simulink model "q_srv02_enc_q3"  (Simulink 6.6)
settings: Solver=FixedStepDiscrete  StartTime=0.0  StopTime=inf  FixedStep=0.002  RelTol=1e-3  AbsTol=1e-6
undefined symbols (not defined in the file or in its folder): HIL, qc_get_step_size
libraries: quarc_library x3, simulink x1

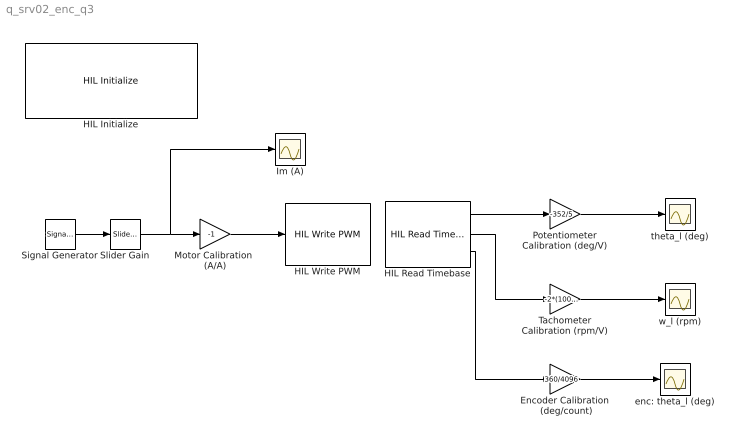
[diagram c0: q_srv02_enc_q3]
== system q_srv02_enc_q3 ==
  Encoder Calibration  (deg/count) : Gain  Gain=360/4096
  HIL Initialize : quarc_library/Data Acquisition/Generic/Configuration/HIL Initialize  object_name=HIL-1  board_type=q3_controlpaq_fw  board_number=0  exclusive=off  active=on  hardware_clocks=[]  clock_modes=[]  set_clock_params_at_start=off  set_clock_params_at_switch_in=off  analog_input_channels=0:1  analog_input_maximums=10  analog_input_minimums=-10  set_analog_input_params_at_start=off  set_analog_input_params_at_switch_in=off  analog_output_channels=[]  analog_output_maximums=[]  analog_output_minimums=[]  initial_analog_outputs=[]  final_analog_outputs=[]  watchdog_analog_outputs=[]  set_analog_output_params_at_start=off  set_analog_output_params_at_switch_in=off  set_analog_outputs_at_start=off  set_analog_outputs_at_switch_in=off  set_analog_outputs_at_terminate=off  set_analog_outputs_at_switch_out=off  set_analog_outputs_on_watchdog=off  digital_input_channels=[0:1]  digital_output_channels=[0]  digital_output_configuration=[]  initial_digital_outputs=0  final_digital_outputs=0  watchdog_digital_outputs=[]  set_digital_output_params_at_start=off  set_digital_output_params_at_switch_in=off  set_digital_outputs_at_start=on  set_digital_outputs_at_switch_in=off  set_digital_outputs_at_terminate=on  set_digital_outputs_at_switch_out=off  set_digital_outputs_on_watchdog=off  encoder_channels=0:2  quadrature=[]  encoder_filter_frequency=[]  initial_encoder_counts=0  set_encoder_params_at_start=off  set_encoder_params_at_switch_in=off  set_encoder_counts_at_start=on  set_encoder_counts_at_switch_in=off  pwm_channels=0:2  pwm_modes=[]  pwm_frequency=[]  pwm_configuration=[]  pwm_alignment=[]  pwm_polarity=[]  pwm_leading_deadband=[]  pwm_trailing_deadband=[]  initial_pwm_outputs=0  final_pwm_outputs=0  watchdog_pwm_outputs=[]  set_pwm_params_at_start=off  set_pwm_params_at_switch_in=off  set_pwm_outputs_at_start=on  set_pwm_outputs_at_switch_in=off  set_pwm_outputs_at_terminate=on  set_pwm_outputs_at_switch_out=off  set_pwm_outputs_on_watchdog=off  other_output_channels=[]  initial_other_outputs=[]  final_other_outputs=[]  watchdog_other_outputs=[]  set_other_outputs_at_start=off  set_other_outputs_at_switch_in=off  set_other_outputs_at_terminate=off  set_other_outputs_at_switch_out=off  set_other_outputs_on_watchdog=off
  HIL Read Timebase : quarc_library/Data Acquisition/Generic/Timebases/HIL Read Timebase  object_name=HIL-1  clock=0  analog_channels=[0,1]  encoder_channels=[0]  digital_channels=[]  other_channels=[]  samples_in_buffer=max(ceil(1/qc_get_step_size), 1)  active=on  vector_output=off  data_type_mode=Inherit via back propagation  encoder_data_type=double  digital_data_type=boolean
  HIL Write PWM : quarc_library/Data Acquisition/Generic/Immediate I//O/HIL Write PWM  object_name=HIL-1  channels=0  sample_time=-1  active=off  vector_input=off
  Im (A) : Scope
  Motor Calibration  (A/A) : Gain  Gain=-1
  Potentiometer Calibration (deg/V) : Gain  Gain=-352/5
  Signal Generator : SignalGenerator
  Slider Gain : simulink/Math Operations/Slider Gain  SystemSampleTime=-1  low=0  gain=0.25  high=0.5
  Tachometer Calibration (rpm/V) : Gain  Gain=-2*(1000/1.5/70)
  enc: theta_l (deg) : Scope
  theta_l (deg) : Scope
  w_l (rpm) : Scope
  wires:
  Signal Generator/1 -> Slider Gain/1
  Slider Gain/1 -> Motor Calibration  (A/A)/1, Im (A)/1
  HIL Read Timebase/1 -> Potentiometer Calibration (deg/V)/1
  Motor Calibration  (A/A)/1 -> HIL Write PWM/1
  Potentiometer Calibration (deg/V)/1 -> theta_l (deg)/1
  HIL Read Timebase/2 -> Tachometer Calibration (rpm/V)/1
  Tachometer Calibration (rpm/V)/1 -> w_l (rpm)/1
  HIL Read Timebase/3 -> Encoder Calibration  (deg/count)/1
  Encoder Calibration  (deg/count)/1 -> enc: theta_l (deg)/1
